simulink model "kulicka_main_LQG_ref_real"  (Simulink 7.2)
libraries: execlib x4

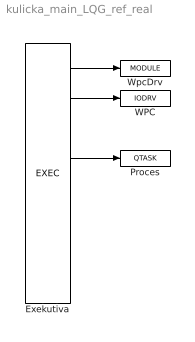
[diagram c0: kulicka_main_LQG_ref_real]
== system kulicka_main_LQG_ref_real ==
  Exekutiva : execlib/EXEC  SystemSampleTime=-1  target=Generic 1ms - Windows CE  tick=0.02  ntick0=1  ntick1=50  ntick2=100  ntick3=1200  pri0=5  pri1=9  pri2=13  pri3=18
  Proces : execlib/QTASK  SystemSampleTime=-1  factor=1  stack=2048  filename=kulicka_proces_LQG_ref_real  MDLOPEN=off
  WPC : execlib/IODRV  classname=WpcDrv  cfgname=WpcDrv.rio  factor=10  stack=10240  pri=3
  WpcDrv : execlib/MODULE
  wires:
  Exekutiva/1 -> WpcDrv/1
  Exekutiva/2 -> WPC/1
  Exekutiva/4 -> Proces/1
